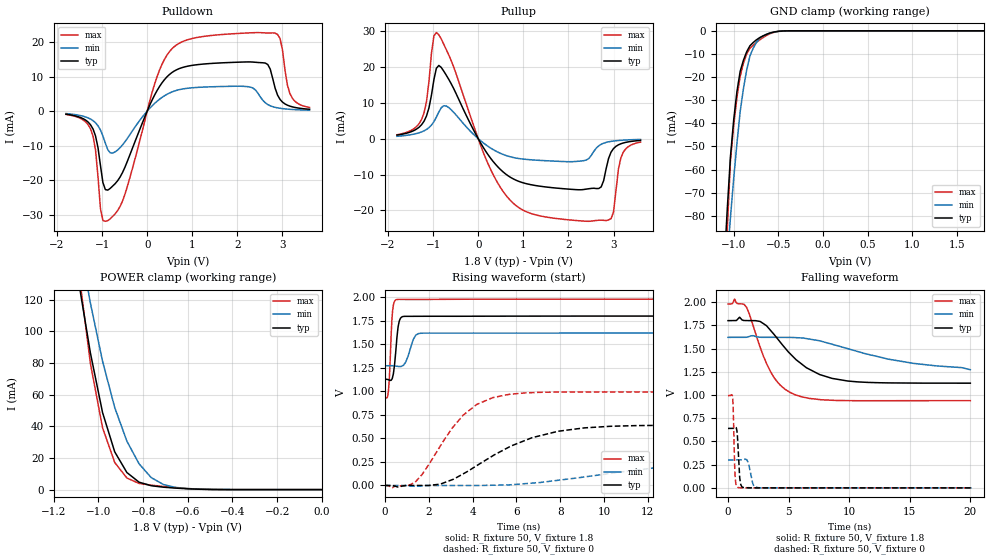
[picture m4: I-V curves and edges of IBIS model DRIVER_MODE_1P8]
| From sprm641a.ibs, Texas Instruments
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|   Model Cell DRIVER_MODE_1P8
|DRIVER_MODE_1P8
[Model]   DRIVER_MODE_1P8
Model_type   I/O
Polarity   Non-Inverting
Enable   Active-Low
Vinl =  0.63
Vinh =  1.17
Cref =  15.0000pF
Rref =  100.0000M
Vref =  0V
Vmeas =  0.9
C_comp   1.111906p   0.9691991p   1.265789p
[Model Spec]
Vinl   0.63   0.63   0.63
Vinh   1.17   1.17   1.17
[Temperature Range]   25   155   -40
[Voltage Range]   1.8   1.62   1.98
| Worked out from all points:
|   slope of the pulldown table from 0 to 0.27 V, typ, clamps not added: 38.3 ohm
|   slope of the pullup table from 0 to 0.27 V, typ, clamps not added: 50.4 ohm
|   GND clamp passes 1 mA (typ) near -0.60 V on its own axis
|   POWER clamp passes 1 mA (typ) near -0.66 V on its own axis
|   rising waveform, R_fixture 50, V_fixture 1.8: 20-80 % time 164ps typ, 290ps min, 119ps max; typ from 1.13 V to 1.8 V
|   rising waveform, R_fixture 50, V_fixture 0: 20-80 % time 3.18ns typ, 6.81ns min, 1.89ns max; typ from 0 V to 0.64 V
|   falling waveform, R_fixture 50, V_fixture 1.8: 20-80 % time 3.22ns typ, 6.76ns min, 2.02ns max; typ from 1.8 V to 1.13 V
|   falling waveform, R_fixture 50, V_fixture 0: 20-80 % time 156ps typ, 284ps min, 116ps max; typ from 0.64 V to 0 V
| Nom Voltages:
|   VDD=1.2, VDDS=1.8, VSS=0
| Min Voltages:
|   VDD=1.08, VDDS=1.62, VSS=0
| Max Voltages:
|   VDD=1.32, VDDS=1.98, VSS=0
[POWER_clamp]
|   voltage   I(typ)   I(min)   I(max)
-1.8V     884.3mA    853.3mA    1.248A
-1.091V   133.1mA    160.5mA    140.6mA
-1.073V   117.6mA    146.3mA    120.4mA
-1.036V   86.44mA    117.9mA    79.83mA
-981.8mV  48.72mA    81.13mA    39.14mA
-927.3mV  23.87mA    51.84mA    17.13mA
-872.7mV  10.78mA    30.59mA    7.315mA
-818.2mV  4.685mA    16.28mA    3.914mA
-763.6mV  2.445mA    7.569mA    2.812mA
-709.1mV  1.528mA    3.185mA    1.975mA
-545.5mV  218.1uA    300.1uA    266.9uA
0V        10.98pA    1.501nA    339.7fA
[Pulldown]
|   voltage   I(typ)   I(min)   I(max)
-1.8V     -902.8uA   -704.1uA   -963.2uA
-1.255V   -3.986mA   -2.313mA   -5.172mA
-1.145V   -7.184mA   -3.376mA   -11.23mA
-1.036V   -15.72mA   -5.465mA   -28.24mA
-927.3mV  -22.72mA   -9.309mA   -31.89mA
-545.5mV  -17.73mA   -9.758mA   -25.97mA
218.2mV   5.927mA    2.847mA    9.932mA
709.1mV   12.29mA    6.199mA    19.63mA
2.618V    13.9mA     2.408mA    22.63mA
2.836V    6.636mA    1.092mA    22.55mA
3.164V    1.438mA    516.7uA    5.106mA
3.6V      532.7uA    256uA      1.039mA
[Pullup]
|   voltage   I(typ)   I(min)   I(max)
-1.8V     1.001mA    655.2uA    1.101mA
-1.255V   3.893mA    1.881mA    5.37mA
-1.091V   8.619mA    3.081mA    15.98mA
-927.3mV  19.6mA     5.997mA    29.54mA
-709.1mV  17.7mA     9.103mA    24.85mA
272.7mV   -5.409mA   -2.589mA   -8.487mA
981.8mV   -12.24mA   -5.663mA   -19.83mA
2.345V    -14.15mA   -6.107mA   -22.96mA
2.673V    -13.88mA   -1.993mA   -22.71mA
2.945V    -3.766mA   -756.6uA   -22.26mA
3.164V    -1.417mA   -456.3uA   -5.348mA
3.6V      -495.8uA   -216.4uA   -962.8uA
[GND_clamp]
|   voltage   I(typ)   I(min)   I(max)
-1.8V     -722.8mA   -541.3mA   -1.24A
-1.109V   -103.2mA   -119.1mA   -124.9mA
-1.073V   -77.59mA   -99.55mA   -86.64mA
-1.036V   -54.39mA   -80.71mA   -56.16mA
-1V       -38.52mA   -63.93mA   -40.94mA
-963.6mV  -26.22mA   -48.65mA   -28.77mA
-927.3mV  -17.5mA    -34.87mA   -19.65mA
-890.9mV  -12.72mA   -24.96mA   -14.02mA
-818.2mV  -6.461mA   -10.87mA   -7.533mA
-709.1mV  -2.938mA   -3.201mA   -3.9mA
-454.5mV  -76.85uA   -139.1uA   -83.47uA
1.8V      10.98pA    88.96nA    62.17fA
[Ramp]
| variable   typ   min   max
dV/dt_f 0.42563308/3.3077055n 0.21980569/6.9993541n 0.65627198/2.0670687n
dV/dt_r 0.39448084/3.2303512n 0.18569157/6.939164n   0.6116978/1.9277963n
R_load = 50
[Rising Waveform]
R_fixture = 50
V_fixture = 1.8
V_fixture_min = 1.62
V_fixture_max = 1.98
|   time   V(typ)   V(min)   V(max)
0s        1.127V     1.272V     938.7mV
162.9ps   1.124V     1.273V     1.001V
336.8ps   1.134V     1.272V     1.804V
418.8ps   1.238V     1.271V     1.944V
554.7ps   1.579V     1.267V     1.976V
657.7ps   1.746V     1.264V     1.977V
764.7ps   1.789V     1.266V     1.977V
1.295ns   1.797V     1.55V      1.977V
1.644ns   1.798V     1.618V     1.977V
20.01ns   1.8V       1.62V      1.98V
[Rising Waveform]
R_fixture = 50
V_fixture = 0
V_fixture_min = 0
V_fixture_max = 0
|   time   V(typ)   V(min)   V(max)
0s        0V         0V         0V
321ps     0V         0V         -25.28mV
1.385ns   0V         -8.757mV   34.76mV
2.523ns   13.72mV    0V         416.4mV
3.58ns    124.2mV    0V         748.7mV
4.924ns   315.5mV    2.771mV    933.4mV
6.717ns   508mV      25.06mV    986.4mV
9.103ns   612mV      90.51mV    994.1mV
14.45ns   640.4mV    234.2mV    993.6mV
20.11ns   639.8mV    300.5mV    993.5mV
[Falling Waveform]
R_fixture = 50
V_fixture = 1.8
V_fixture_min = 1.62
V_fixture_max = 1.98
|   time   V(typ)   V(min)   V(max)
0s        1.8V       1.62V      1.98V
541.3ps   1.799V     1.62V      2.032V
1.522ns   1.801V     1.621V     1.946V
2.653ns   1.791V     1.621V     1.515V
3.45ns    1.706V     1.62V      1.265V
4.368ns   1.559V     1.62V      1.099V
5.498ns   1.396V     1.618V     1.004V
7.535ns   1.221V     1.584V     950.9mV
9.889ns   1.15V      1.499V     939.1mV
20.01ns   1.127V     1.272V     938.9mV
[Falling Waveform]
R_fixture = 50
V_fixture = 0
V_fixture_min = 0
V_fixture_max = 0
|   time   V(typ)   V(min)   V(max)
0s        639.8mV    300.5mV    993.5mV
391.7ps   639.5mV    300mV      955.9mV
587.4ps   648.1mV    299.9mV    123.1mV
736.1ps   614.8mV    300mV      11.36mV
828.7ps   440.6mV    300.1mV    3.593mV
999ps     71.45mV    300.6mV    0V
1.252ns   4.794mV    304.3mV    0V
2.082ns   0V         33.09mV    0V
2.618ns   0V         0V         0V
20.11ns   0V         0V         0V
